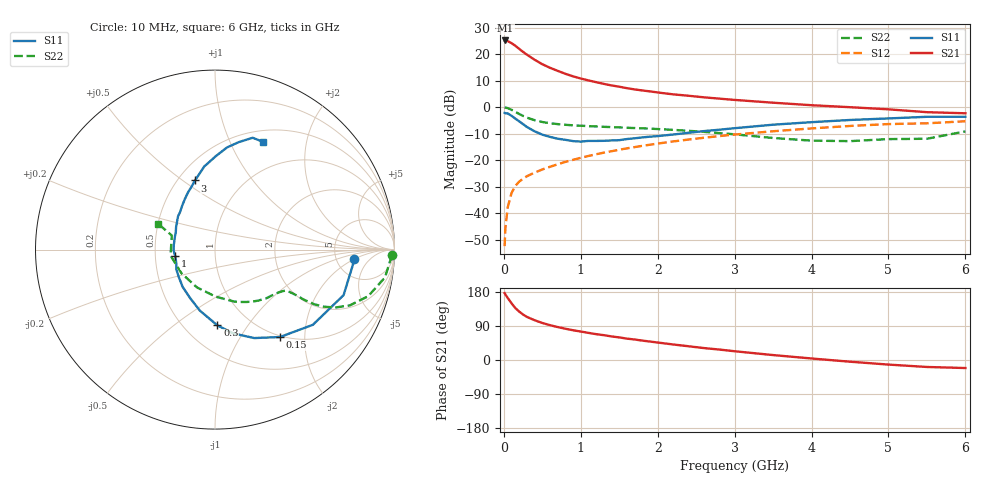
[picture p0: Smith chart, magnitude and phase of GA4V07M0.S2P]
! Infineon Technologies  Discrete & RF Semiconductors
! BF775
! Si NPN RF Bipolar Junction Transistor in SOT23
! VCE = 4 V  IC = 7 mA
! Common Emitter S-Parameters:  May  1996
# GHz  S  MA  R  50
!  f  S11  S21  S12  S22
! GHz  MAG  ANG  MAG  ANG  MAG  ANG  MAG  ANG
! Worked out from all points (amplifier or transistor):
!   36 points, 10 MHz to 6 GHz, reference 50 ohm
!   highest |S21| = 25.1 dB at 20 MHz (marker M1)
!   |S21| within 3 dB of that: start of sweep to 192.3 MHz
!   unconditionally stable (mu >= 1): 696.7 MHz to 3.243 GHz
!   at 250 MHz: K = 0.57, MSG = 23.9 dB, |S12| = -27.0 dB
!   at 1.4 GHz: K = 1.12, MAG = 10.3 dB, |S12| = -16.6 dB
!   at 6 GHz: K = 0.94, MSG = 1.5 dB, |S12| = -5.3 dB
!   S11 on the Smith chart (normalised r, x): 10 MHz: 7.47, -2.06; 150 MHz: 0.98, -1.51; 300 MHz: 0.71, -0.73; 1 GHz: 0.64, -0.05; 3 GHz: 0.61, +0.56; 6 GHz: 0.63, +1.33
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0.01  0.7789 -4.0  17.96 176.6  0.0024 84.6  0.9879 -1.8
0.02  0.7689 -8.0  18.04 173.1  0.0052 84.5  0.9775 -3.8
0.05  0.76 -19.5  17.55 163.7  0.0129 80.1  0.9597 -9.3
0.1  0.6878 -37.5  16.04 149.7  0.0241 72.4  0.8923 -16.9
0.15  0.6068 -53.4  14.3 136.8  0.0329 66.5  0.8127 -22.5
0.2  0.5391 -66.1  12.51 127.7  0.0395 62.5  0.7422 -25.8
0.25  0.4784 -77.6  10.98 119.9  0.0449 60.6  0.6831 -27.7
0.3  0.4224 -88.2  9.74 113.7  0.0499 59.6  0.6335 -28.8
0.4  0.3504 -103.9  7.817 105.0  0.0584 59.3  0.5678 -29.4
0.5  0.3028 -117.5  6.433 97.7  0.0669 59.7  0.5247 -29.3
0.6  0.2752 -130.9  5.514 91.9  0.0752 60.0  0.4976 -29.4
0.7  0.254 -142.2  4.826 86.9  0.0837 60.9  0.479 -29.6
0.8  0.242 -152.9  4.246 82.5  0.093 61.2  0.465 -29.8
1  0.2242 -170.3  3.462 75.1  0.1109 61.4  0.4464 -31.1
1.1  0.231 -179.0  3.191 71.6  0.1201 61.4  0.4383 -32.1
1.6  0.2504 150.0  2.275 56.4  0.1672 59.5  0.4084 -38.5
2.2  0.3047 127.0  1.742 41.0  0.2257 54.8  0.3733 -49.5
3  0.4011 106.1  1.367 23.1  0.3043 46.5  0.3074 -70.1
3.5  0.4667 97.4  1.212 13.0  0.3511 40.4  0.2621 -89.2
4.5  0.573 83.3  0.997 -4.5  0.4417 27.5  0.2287 -144.7
5.5  0.6574 71.4  0.803 -18.4  0.4958 12.7  0.2535 161.9
6  0.6575 66.2  0.766 -21.2  0.5419 8.6  0.3493 155.5
